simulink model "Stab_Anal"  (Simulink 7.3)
settings: Solver=ode45  StartTime=0.0  StopTime=10  RelTol=1e-3
InitFcn:
  | init
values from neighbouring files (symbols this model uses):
  calfa = cos(alfa0*d2r)    [init.m]
  d2r = pi/180    (= 0.0174532925199)    [init.m]    (also in robust.m)
  ge = 32.174    [init.m]
  r2d = 180/pi    (= 57.2957795131)    [init.m]    (also in robust.m)
  salfa = sin(alfa0*d2r)    [init.m]
  Thet0 = 27.69    [init.m]
  V0 = 24675.1    [init.m]
  x0 = [0 0 -2 -2 0 0 18 0 0 0]'*d2r    [init.m]
undefined symbols (not defined in the file or in its folder): As, Bs, Cs, Ds, Kmix, Kpr, Kq

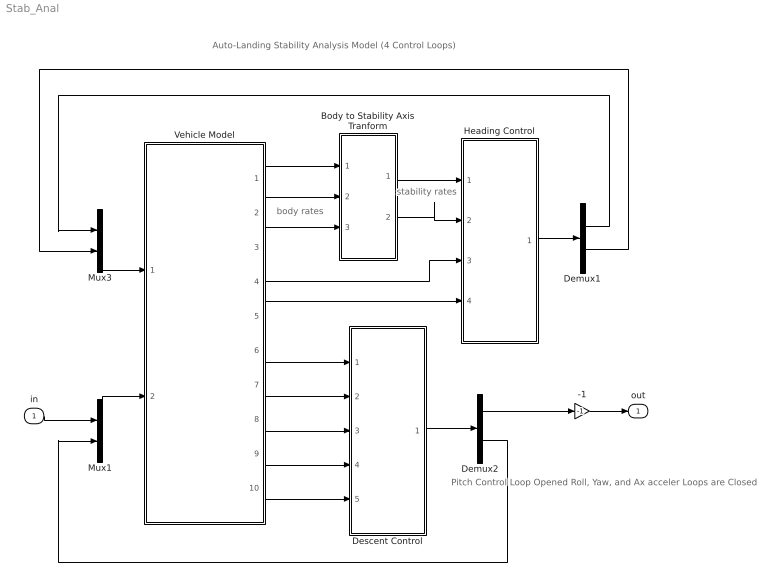
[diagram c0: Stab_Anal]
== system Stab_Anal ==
  note: Auto-Landing Stability Analysis Model (4 Control Loops)
  note: body rates
  note: stability rates
  note: Pitch Control Loop Opened Roll, Yaw, and Ax acceler Loops are Closed
  in : Inport  OutDataType=sfix(16)  OutScaling=2^0
  -1 : Gain  Gain=-1  ParameterDataType=sfix(16)  ParameterScaling=2^0  OutDataType=sfix(16)  OutScaling=2^0
  Body to Stability Axis Tranform : Subsystem
  Demux1 : Demux  Outputs=2
  Demux2 : Demux  Outputs=2
  Descent Control : Subsystem
  Heading Control : Subsystem
  Mux1 : Mux  Inputs=2
  Mux3 : Mux  Inputs=2
  Vehicle Model : Subsystem
  out : Outport  OutDataType=sfix(16)  OutScaling=2^0
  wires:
  Vehicle Model/6(theta) -> Descent Control/1(theta)
  Vehicle Model/7(q) -> Descent Control/2(q)
  Vehicle Model/8(dH) -> Descent Control/3(dH)
  Vehicle Model/9(dV) -> Descent Control/4(dV)
  Vehicle Model/10(Nz) -> Descent Control/5(Nz)
  Vehicle Model/3(r) -> Body to Stability Axis Tranform/3(r_b)
  Vehicle Model/2(p) -> Body to Stability Axis Tranform/2(p_b)
  Vehicle Model/1(phi) -> Body to Stability Axis Tranform/1(phi)
  Body to Stability Axis Tranform/1(p_s) -> Heading Control/1(ps)
  Body to Stability Axis Tranform/2(r_s) -> Heading Control/2(rs)
  Vehicle Model/5(Vcr) -> Heading Control/4(Vcr)
  Vehicle Model/4(Ny) -> Heading Control/3(Ny)
  Heading Control/1((dP,dR)) -> Demux1/1
  Mux3/1 -> Vehicle Model/1("(dP, dR)")
  Descent Control/1((dQ,dV)) -> Demux2/1
  Mux1/1 -> Vehicle Model/2("(dQ, dV)")
  -1/1 -> out/1
  Demux2/2 -> Mux1/2
  Demux1/1 -> Mux3/1
  in/1 -> Mux1/1
  Demux2/1 -> -1/1
  Demux1/2 -> Mux3/2

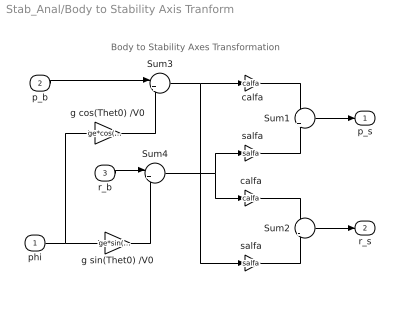
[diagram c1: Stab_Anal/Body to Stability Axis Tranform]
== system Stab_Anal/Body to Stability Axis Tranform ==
  note: Body to Stability Axes Transformation
  phi : Inport  OutDataType=sfix(16)  OutScaling=2^0
  p_b : Inport  Port=2  OutDataType=sfix(16)  OutScaling=2^0
  r_b : Inport  Port=3  OutDataType=sfix(16)  OutScaling=2^0
  Sum1 : Sum  Inputs=+|+  OutDataType=sfix(16)  OutScaling=2^0
  Sum2 : Sum  Inputs=+|-  OutDataType=sfix(16)  OutScaling=2^0
  Sum3 : Sum  Inputs=|++  OutDataType=sfix(16)  OutScaling=2^0
  Sum4 : Sum  Inputs=|+-  OutDataType=sfix(16)  OutScaling=2^0
  calfa : Gain  Gain=calfa  ParameterDataType=sfix(16)  ParameterScaling=2^0  OutDataType=sfix(16)  OutScaling=2^0
  "calfa " : Gain  Gain=calfa  ParameterDataType=sfix(16)  ParameterScaling=2^0  OutDataType=sfix(16)  OutScaling=2^0
  g cos(Thet0) /V0 : Gain  Gain=ge*cos(Thet0*d2r)/V0  ParameterDataType=sfix(16)  ParameterScaling=2^0  OutDataType=sfix(16)  OutScaling=2^0
  g sin(Thet0) /V0 : Gain  Gain=ge*sin(Thet0*d2r)/V0  ParameterDataType=sfix(16)  ParameterScaling=2^0  OutDataType=sfix(16)  OutScaling=2^0
  salfa : Gain  Gain=salfa  ParameterDataType=sfix(16)  ParameterScaling=2^0  OutDataType=sfix(16)  OutScaling=2^0
  "salfa " : Gain  Gain=salfa  ParameterDataType=sfix(16)  ParameterScaling=2^0  OutDataType=sfix(16)  OutScaling=2^0
  p_s : Outport  OutDataType=sfix(16)  OutScaling=2^0
  r_s : Outport  Port=2  OutDataType=sfix(16)  OutScaling=2^0
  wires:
  Sum1/1 -> p_s/1
  Sum2/1 -> r_s/1
  p_b/1 -> Sum3/1
  r_b/1 -> Sum4/1
  g cos(Thet0) /V0/1 -> Sum3/2
  g sin(Thet0) /V0/1 -> Sum4/2
  phi/1 -> g cos(Thet0) /V0/1, g sin(Thet0) /V0/1
  Sum4/1 -> "calfa "/1, salfa/1
  Sum3/1 -> "salfa "/1, calfa/1
  calfa/1 -> Sum1/1
  salfa/1 -> Sum1/2
  "calfa "/1 -> Sum2/1
  "salfa "/1 -> Sum2/2

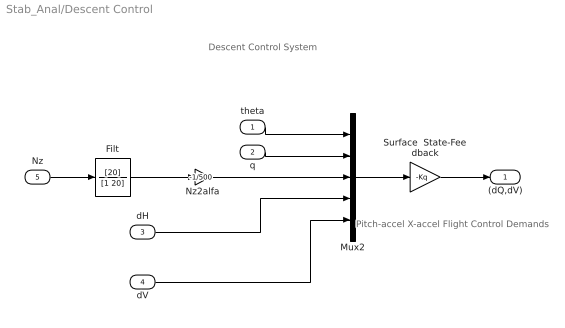
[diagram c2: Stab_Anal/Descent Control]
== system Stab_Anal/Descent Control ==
  note: Pitch-accel X-accel Flight Control Demands
  note: Descent Control System
  theta : Inport
  q : Inport  Port=2
  dH : Inport  Port=3
  dV : Inport  Port=4
  Nz : Inport  Port=5
  Filt : TransferFcn  Numerator=[20]  Denominator=[1 20]
  Mux2 : Mux  Inputs=5
  Nz2alfa : Gain  Gain=-1/500  ParameterDataType=sfix(16)  ParameterScaling=2^0  OutDataType=sfix(16)  OutScaling=2^0
  Surface  State-Feedback : Gain  Gain=-Kq  Multiplication=Matrix(K*u)  ParameterDataType=sfix(16)  ParameterScaling=2^0  OutDataType=sfix(16)  OutScaling=2^0
  (dQ,dV) : Outport
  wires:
  theta/1 -> Mux2/1
  q/1 -> Mux2/2
  dH/1 -> Mux2/4
  dV/1 -> Mux2/5
  Nz/1 -> Filt/1
  Mux2/1 -> Surface  State-Feedback/1
  Surface  State-Feedback/1 -> (dQ,dV)/1
  Nz2alfa/1 -> Mux2/3
  Filt/1 -> Nz2alfa/1

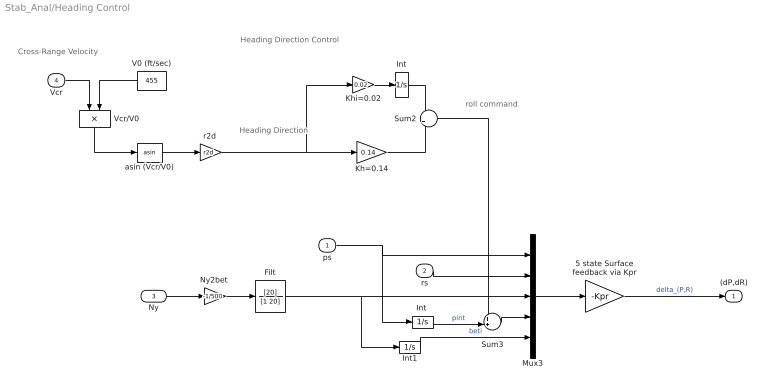
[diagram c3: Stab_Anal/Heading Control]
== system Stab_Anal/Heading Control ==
  note: Heading Direction Control
  note: roll command
  note: Heading Direction
  note: Cross-Range Velocity
  ps : Inport  OutDataType=sfix(16)  OutScaling=2^0
  rs : Inport  Port=2  OutDataType=sfix(16)  OutScaling=2^0
  Ny : Inport  Port=3
  Vcr : Inport  Port=4  OutDataType=sfix(16)  OutScaling=2^0
  5 state Surface feedback via Kpr : Gain  Gain=-Kpr  Multiplication=Matrix(K*u)  ParameterDataType=sfix(16)  ParameterScaling=2^0  OutDataType=sfix(16)  OutScaling=2^0
  Filt : TransferFcn  Numerator=[20]  Denominator=[1 20]
  Int : Integrator
  "Int " : Integrator
  Int1 : Integrator
  Kh=0.14 : Gain  Gain=0.14  ParameterDataType=sfix(16)  ParameterScaling=2^0  OutDataType=sfix(16)  OutScaling=2^0
  Khi=0.02 : Gain  Gain=0.02  ParameterDataType=sfix(16)  ParameterScaling=2^0  OutDataType=sfix(16)  OutScaling=2^0
  Mux3 : Mux  Inputs=5
  "Ny2bet " : Gain  Gain=-1/500  ParameterDataType=sfix(16)  ParameterScaling=2^0  OutDataType=sfix(16)  OutScaling=2^0
  Sum2 : Sum  OutDataType=sfix(16)  OutScaling=2^0
  Sum3 : Sum  Inputs=++|  OutDataType=sfix(16)  OutScaling=2^0
  V0 (ft/sec) : Constant  Value=455  OutDataType=sfix(16)  OutScaling=2^0
  Vcr/V0 : Product  Inputs=*/  OutDataType=sfix(16)  OutScaling=2^0
  asin (Vcr/V0) : Trigonometry  Operator=asin
  "r2d " : Gain  Gain=r2d  ParameterDataType=sfix(16)  ParameterScaling=2^0  OutDataType=sfix(16)  OutScaling=2^0
  (dP,dR) : Outport  OutDataType=sfix(16)  OutScaling=2^0
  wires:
  Vcr/1 -> Vcr/V0/1
  Sum2/1 -> Sum3/1
  Int/1 -> Sum2/1
  Kh=0.14/1 -> Sum2/2
  Khi=0.02/1 -> Int/1
  "r2d "/1 -> Kh=0.14/1, Khi=0.02/1
  Vcr/V0/1 -> asin (Vcr/V0)/1
  asin (Vcr/V0)/1 -> "r2d "/1
  V0 (ft/sec)/1 -> Vcr/V0/2
  Mux3/1 -> 5 state Surface feedback via Kpr/1
  5 state Surface feedback via Kpr/1 -> (dP,dR)/1  "delta_(P,R)"
  rs/1 -> Mux3/2
  ps/1 -> "Int "/1, Mux3/1
  Int1/1 -> Mux3/5  "beti"
  Sum3/1 -> Mux3/4
  "Int "/1 -> Sum3/2  "pint"
  "Ny2bet "/1 -> Filt/1
  Ny/1 -> "Ny2bet "/1
  Filt/1 -> Int1/1, Mux3/3

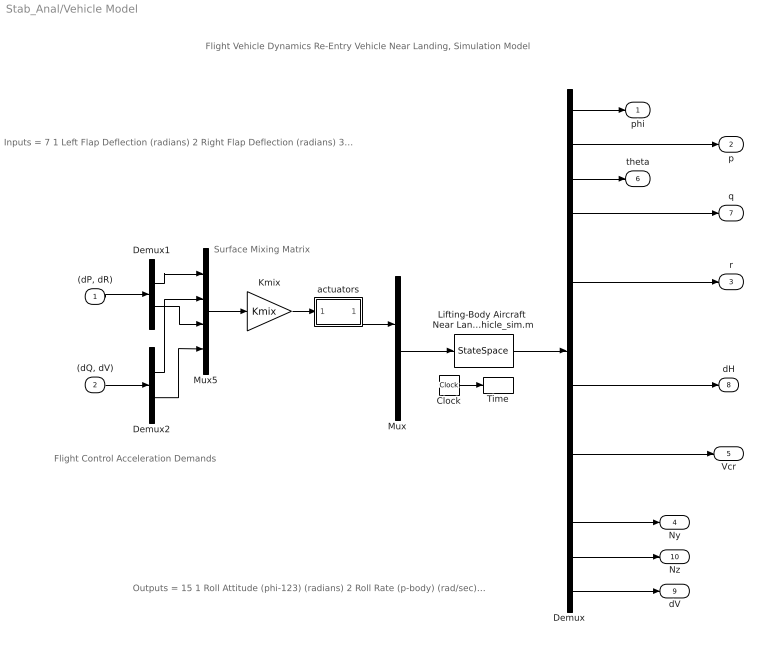
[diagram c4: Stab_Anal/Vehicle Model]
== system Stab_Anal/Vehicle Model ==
  note: Flight Vehicle Dynamics Re-Entry Vehicle Near Landing, Simulation Model
  note: Surface Mixing Matrix
  note: Inputs = 7 1 Left Flap Deflection (radians) 2 Right Flap Deflection (radians) 3 Left Rudder Deflection (radians) 4 Right Rudder Deflection (radians) 5 Body-Flap Deflection (radians) 6 Rudder Deflection (radians) 7 Wind Gust Azim & Elev Angles =(45, 90) (deg)
  note: Outputs = 15 1 Roll Attitude (phi-123) (radians) 2 Roll Rate (p-body) (rad/sec) 3 Pitch Attitude (thet-123) (radians) 4 Pitch Rate (q-body) (rad/sec) 5 Yaw Attitude (psi-123) (radians) 6 Yaw Rate (r-body) (rad/sec) 7 Angle of attack, alfa, (radians) 8 Angle of sideslip, beta, (radian) 9 Change in Altitude, delta-h, (feet) 10 Forward Acceleration (V-dot) (ft/sec) 11 Cross Range Velocity (Vcr) (ft/sec) 12 Accelerom # 1, (along X), (ft/sec^2) Translat. Acceler 13 Accelerom # 2, (along Y), (ft/sec^2) Translat. Acceler 14 Accelerom # 3, (along Z), (ft/sec^2) Translat. Acceler 15 Change in Velocity (delta-V) (ft/sec)
  note: Flight Control Acceleration Demands
  "(dP, dR)" : Inport  OutDataType=sfix(16)  OutScaling=2^0
  "(dQ, dV)" : Inport  Port=2  OutDataType=sfix(16)  OutScaling=2^0
  Clock : Clock
  Demux : Demux  Outputs=15
  Demux1 : Demux  Outputs=2
  Demux2 : Demux  Outputs=2
  Kmix : Gain  Gain=Kmix  Multiplication=Matrix(K*u)  ParameterDataType=sfix(16)  ParameterScaling=2^0  OutDataType=sfix(16)  OutScaling=2^0
  "Lifting-Body Aircraft  Near Landing,  Simulation Model  from file vehicle_sim.m" : StateSpace  A=As  B=Bs  C=Cs  D=Ds  X0=x0
  Mux : Mux  Inputs=[7,1]
  Mux5 : Mux
  Time : ToWorkspace  VariableName=time  SampleTime=-1  SaveFormat=Array
  actuators : Subsystem
  phi : Outport  OutDataType=sfix(16)  OutScaling=2^0
  p : Outport  Port=2  OutDataType=sfix(16)  OutScaling=2^0
  r : Outport  Port=3  OutDataType=sfix(16)  OutScaling=2^0
  Ny : Outport  Port=4  OutDataType=sfix(16)  OutScaling=2^0
  Vcr : Outport  Port=5  OutDataType=sfix(16)  OutScaling=2^0
  theta : Outport  Port=6  OutDataType=sfix(16)  OutScaling=2^0
  q : Outport  Port=7  OutDataType=sfix(16)  OutScaling=2^0
  dH : Outport  Port=8  OutDataType=sfix(16)  OutScaling=2^0
  dV : Outport  Port=9  OutDataType=sfix(16)  OutScaling=2^0
  Nz : Outport  Port=10  OutDataType=sfix(16)  OutScaling=2^0
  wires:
  Mux/1 -> "Lifting-Body Aircraft  Near Landing,  Simulation Model  from file vehicle_sim.m"/1
  Clock/1 -> Time/1
  "Lifting-Body Aircraft  Near Landing,  Simulation Model  from file vehicle_sim.m"/1 -> Demux/1
  Kmix/1 -> actuators/1(In)
  actuators/1(out) -> Mux/1
  Demux/1 -> phi/1
  Demux/3 -> theta/1
  Demux/2 -> p/1
  Demux/4 -> q/1
  Demux/6 -> r/1
  Demux/9 -> dH/1
  Demux/15 -> dV/1
  Demux/13 -> Ny/1
  Demux/14 -> Nz/1
  Demux/11 -> Vcr/1
  Mux5/1 -> Kmix/1
  Demux1/1 -> Mux5/1
  Demux1/2 -> Mux5/3
  Demux2/1 -> Mux5/2
  Demux2/2 -> Mux5/4
  "(dP, dR)"/1 -> Demux1/1
  "(dQ, dV)"/1 -> Demux2/1

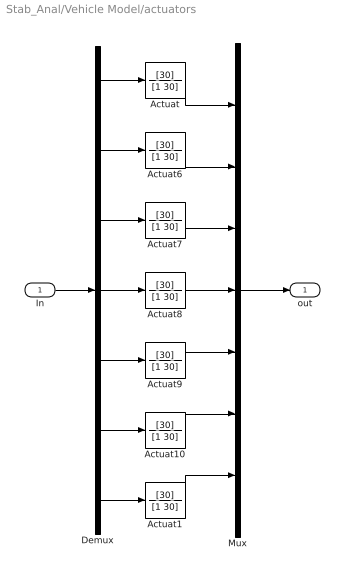
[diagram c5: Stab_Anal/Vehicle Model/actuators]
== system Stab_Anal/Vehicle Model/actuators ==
  In : Inport
  Actuat{,1,6..10} (7 alike) : TransferFcn  Numerator=[30]  Denominator=[1 30]
  Demux : Demux  Outputs=7
  Mux : Mux  Inputs=7
  out : Outport
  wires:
  Actuat10/1 -> Mux/6
  Actuat9/1 -> Mux/5
  Actuat8/1 -> Mux/4
  Actuat7/1 -> Mux/3
  Actuat6/1 -> Mux/2
  Actuat/1 -> Mux/1
  Demux/6 -> Actuat10/1
  Demux/5 -> Actuat9/1
  Demux/4 -> Actuat8/1
  Demux/3 -> Actuat7/1
  Demux/2 -> Actuat6/1
  Demux/1 -> Actuat/1
  Demux/7 -> Actuat1/1
  Actuat1/1 -> Mux/7
  Mux/1 -> out/1
  In/1 -> Demux/1
